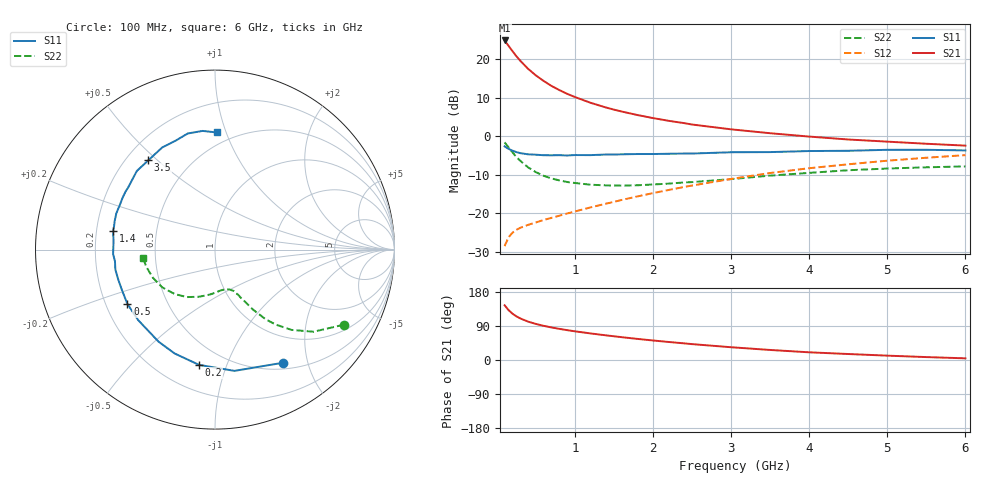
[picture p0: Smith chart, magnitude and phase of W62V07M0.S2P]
! SIEMENS Small Signal Semiconductors
! BFR193W
! Si NPN RF Bipolar Junction Transistor in SOT323
! VCE = 2 V  IC = 7 mA
! Common Emitter S-Parameters:  September  1992
# GHz  S  MA  R  50
!  f  S11  S21  S12  S22
! GHz  MAG  ANG  MAG  ANG  MAG  ANG  MAG  ANG
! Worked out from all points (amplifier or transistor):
!   28 points, 100 MHz to 6 GHz, reference 50 ohm
!   highest |S21| = 24.8 dB at 100 MHz (marker M1)
!   |S21| within 3 dB of that: start of sweep to 209.5 MHz
!   unconditionally stable (mu >= 1): 1.094 GHz to 2.587 GHz
!   at 300 MHz: K = 0.46, MSG = 21.7 dB, |S12| = -23.8 dB
!   at 1.5 GHz: K = 1.06, MAG = 10.4 dB, |S12| = -17.0 dB
!   at 6 GHz: K = 0.92, MSG = 1.2 dB, |S12| = -4.9 dB
!   lowest NFmin = 1.20 dB at 450 MHz
!   S11 on the Smith chart (normalised r, x): 100 MHz: 0.59, -1.62; 200 MHz: 0.36, -0.80; 500 MHz: 0.29, -0.26; 1.4 GHz: 0.27, +0.08; 3.5 GHz: 0.29, +0.47; 6 GHz: 0.41, +0.93
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0.1  0.7365 -58.8  17.35 144.4  0.0375 62.7  0.8315 -30.2
0.15  0.6843 -80.9  14.79 131.8  0.0489 54.7  0.7149 -39.8
0.2  0.6482 -97.9  12.64 122.3  0.0559 49.4  0.6179 -46.4
0.25  0.621 -111.2  10.88 115.3  0.0611 46.6  0.5374 -51.0
0.3  0.6017 -121.5  9.481 109.8  0.0648 45.0  0.4795 -54.0
0.4  0.581 -137.4  7.455 101.3  0.0708 44.2  0.3943 -57.7
0.5  0.5743 -148.2  6.12 95.2  0.0761 45.0  0.3412 -59.8
0.6  0.5654 -156.5  5.181 90.2  0.082 46.5  0.306 -61.7
0.7  0.5643 -163.0  4.469 85.9  0.0872 48.2  0.2829 -62.9
0.8  0.5662 -168.7  3.952 82.2  0.0931 49.9  0.2668 -64.5
0.9  0.5611 -173.3  3.532 78.8  0.0994 51.6  0.2543 -65.5
1  0.5683 -177.5  3.209 75.7  0.1055 53.3  0.247 -67.1
1.2  0.5671 175.5  2.703 70.1  0.1193 55.8  0.2345 -70.8
1.4  0.5772 169.6  2.345 65.0  0.1333 57.9  0.2301 -74.4
1.8  0.5858 159.8  1.876 55.7  0.1654 60.5  0.2307 -82.9
2.2  0.5907 150.5  1.579 47.6  0.2004 61.5  0.2424 -91.2
2.5  0.5945 144.7  1.413 41.9  0.2288 61.3  0.2536 -97.5
3  0.6178 134.8  1.224 33.7  0.2787 59.6  0.2772 -108.6
3.5  0.6208 126.8  1.09 26.5  0.3327 56.6  0.3077 -120.7
4.5  0.6455 109.8  0.904 15.8  0.4313 48.2  0.3612 -144.3
5.5  0.6649 96.0  0.796 7.7  0.5245 38.7  0.3943 -165.8
6  0.6526 89.0  0.753 4.4  0.567 33.5  0.4049 -173.6
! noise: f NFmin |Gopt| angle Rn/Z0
0.45  1.2  0.24  125  0.12
0.9  1.25  0.36  154  0.11
1.8  2  0.55  -156  0.13
